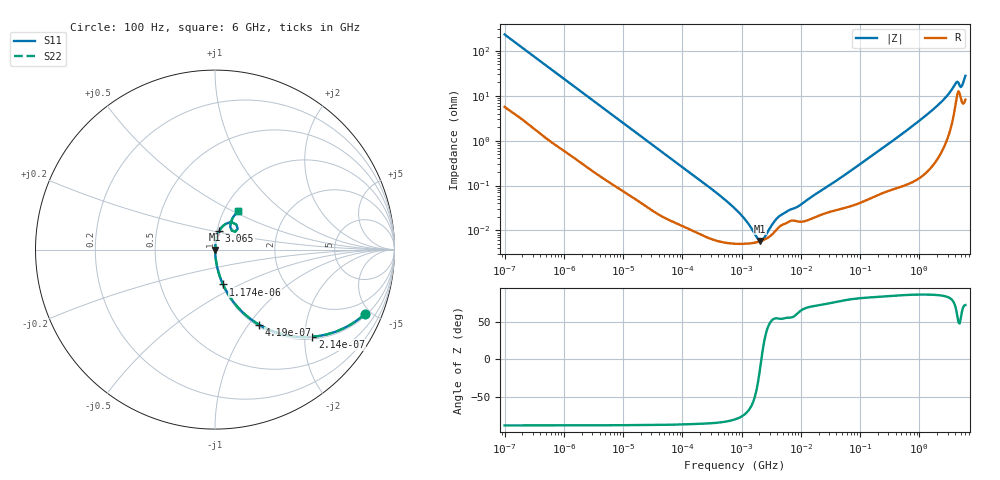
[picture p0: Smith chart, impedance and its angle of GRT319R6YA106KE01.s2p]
!Murata Part Number: GRT319R6YA106KE01
!These Parameters are Measured in Series Mode Connection
!Data Generated on Jun 19, 2026
!  o--ll--o
!Port1  Port2
!  o------o
!Operation Temp=25[degC], DC Bias Voltage=0[V]
!Freq. Start=100[Hz] Stop=6[GHz] 401[Steps]
# Hz S RI R 50
!Freq.(Hz) S11(Real) S11(Imag) S21(Real) S21(Imag) S12(Real) S12(Imag) S22(Real) S22(Imag)
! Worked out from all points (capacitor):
!   401 points, 100 Hz to 6 GHz, reference 50 ohm
!   read as one part in series: C = 6.87 uF near 109 Hz
!   lowest |Z| = 5.83 mohm at 2.074 MHz (marker M1)
!   series resonance near 2.157 MHz, so ESL is about 790 pH
!   S11 on the Smith chart (normalised r, x): 100 Hz: 1.11, -4.61; 214 Hz: 1.05, -2.18; 419 Hz: 1.03, -1.13; 1.174 kHz: 1.01, -0.41; 3.065 GHz: 1.02, +0.21; 6 GHz: 1.16, +0.53
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100  0.8358 -0.3585  0.1642 0.3585  0.1642 0.3585  0.8358 -0.3585
214  0.5423 -0.4858  0.4577 0.4858  0.4577 0.4858  0.5423 -0.4858
419  0.2461 -0.4188  0.7539 0.4188  0.7539 0.4188  0.2461 -0.4188
686  0.113 -0.3048  0.887 0.3048  0.887 0.3048  0.113 -0.3048
1174  0.0445 -0.194  0.9555 0.194  0.9555 0.194  0.0445 -0.194
2008  0.0172 -0.1179  0.9828 0.1179  0.9828 0.1179  0.0172 -0.1179
6433  0.00254 -0.0381  0.9975 0.0381  0.9975 0.0381  0.00254 -0.0381
40335  0.000264 -0.00631  0.9997 0.00631  0.9997 0.00631  0.000264 -0.00631
316350  6.42e-05 -0.000823  0.9999 0.000823  0.9999 0.000823  6.42e-05 -0.000823
774597  5.07e-05 -0.000302  0.9999 0.000302  0.9999 0.000302  5.07e-05 -0.000302
1516199  5.23e-05 -9e-05  0.9999 9e-05  0.9999 9e-05  5.23e-05 -9e-05
2074311  5.75e-05 -9.8e-06  0.9999 9.8e-06  0.9999 9.8e-06  5.75e-05 -9.8e-06
2837864  7.02e-05 6.98e-05  0.9999 -6.98e-05  0.9999 -6.98e-05  7.02e-05 6.98e-05
4440638  0.000123 0.000173  0.9999 -0.000173  0.9999 -0.000173  0.000123 0.000173
9090158  0.000158 0.000307  0.9998 -0.000307  0.9998 -0.000307  0.000158 0.000307
1.555665e7  0.000186 0.000542  0.9998 -0.000542  0.9998 -0.000542  0.000186 0.000542
3.124326e8  0.000846 0.00871  0.9992 -0.00871  0.9992 -0.00871  0.000846 0.00871
1.431855e9  0.00379 0.0403  0.9962 -0.0403  0.9962 -0.0403  0.00379 0.0403
3.065283e9  0.0226 0.1018  0.9774 -0.1018  0.9774 -0.1018  0.0226 0.1018
4.193612e9  0.0973 0.1505  0.9027 -0.1505  0.9027 -0.1505  0.0973 0.1505
5.245841e9  0.085 0.1268  0.915 -0.1268  0.915 -0.1268  0.085 0.1268
6e9  0.1278 0.214  0.8722 -0.214  0.8722 -0.214  0.1278 0.214
